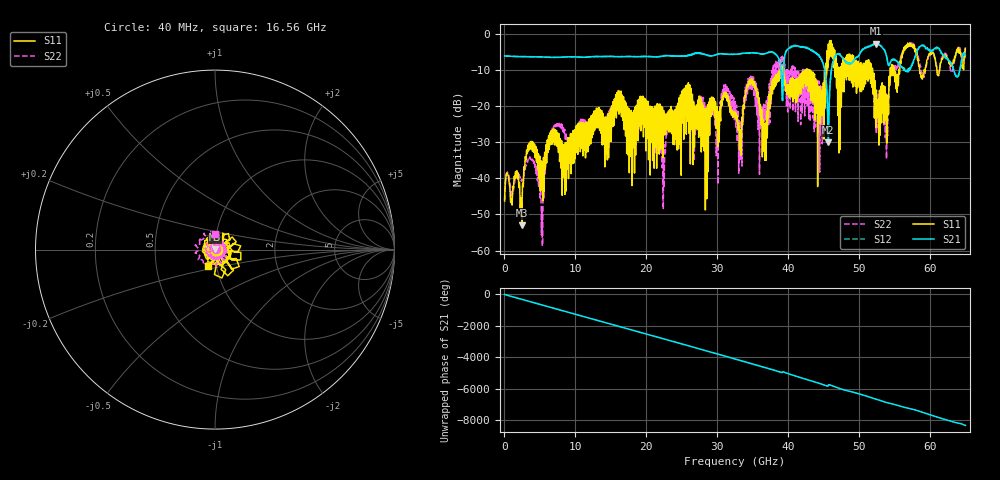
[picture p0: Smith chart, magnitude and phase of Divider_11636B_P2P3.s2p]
! Created Tue Jul 15 20:13:26 2008
# hz S ma R 50
! 2 Port Network Data from blockName block
! freq  magS11  angS11  magS21  angS21  magS12  angS12  magS22  angS22
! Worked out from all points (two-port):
!   1601 points, 40 MHz to 65 GHz, reference 50 ohm
!   highest |S21| = -2.62 dB at 52.37 GHz (marker M1); lowest = -30.0 dB at 45.67 GHz (marker M2)
!   |S21| within 3 dB of the highest: 32.25 GHz to 38.27 GHz (6.024 GHz wide, 17.1 % of centre); 39.57 GHz to 44.18 GHz (4.61 GHz wide, 11 % of centre)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
!   lowest |S11| = -53.0 dB at 2.476 GHz (marker M3), VSWR 1.00, Z = 50.2 + j0.162 ohm
!   |S11| at or under -10 dB: start of sweep to 38.93 GHz; 39.31 GHz to 42.42 GHz (3.113 GHz wide, 7.62 % of centre); 51.92 GHz to 54.4 GHz (2.477 GHz wide, 4.66 % of centre)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
!   |S22| runs from -58.8 to -2.3 dB; largest |S21 - S12| = 0.062
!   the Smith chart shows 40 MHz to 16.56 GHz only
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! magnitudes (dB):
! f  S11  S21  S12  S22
! 40 MHz  -46.3  -6.0  -6.1  -46.1
! 2.476 GHz  -53.0  -6.2  -6.2  -40.4
! 3.613 GHz  -31.9  -6.3  -6.3  -34.1
! 5.318 GHz  -36.2  -6.3  -6.3  -48.1
! 6.698 GHz  -30.6  -6.4  -6.4  -27.3
! 10.88 GHz  -31.6  -6.4  -6.4  -25.7
! 16.16 GHz  -22.2  -6.3  -6.2  -21.1
! 21.72 GHz  -20.0  -6.3  -6.3  -27.0
! 25.37 GHz  -15.0  -6.0  -6.1  -19.3
! 32.52 GHz  -22.2  -5.6  -5.6  -19.2
! 33.33 GHz  -29.3  -5.4  -5.4  -27.4
! 34.92 GHz  -13.7  -5.2  -5.3  -11.5
! 36.7 GHz  -29.6  -5.5  -5.5  -19.6
! 38.93 GHz  -9.8  -8.8  -8.7  -12.2
! 43.36 GHz  -10.5  -4.4  -4.4  -12.4
! 44.5 GHz  -18.0  -6.4  -6.3  -18.2
! 45.67 GHz  -2.8  -30.0  -30.2  -6.5
! 46.77 GHz  -6.9  -5.7  -5.5  -9.5
! 52.37 GHz  -25.9  -2.6  -2.6  -17.9
! 54.2 GHz  -15.4  -8.7  -8.7  -17.6
! 56.92 GHz  -3.0  -10.5  -9.7  -3.0
! 65 GHz  -3.9  -5.8  -6.7  -3.4
